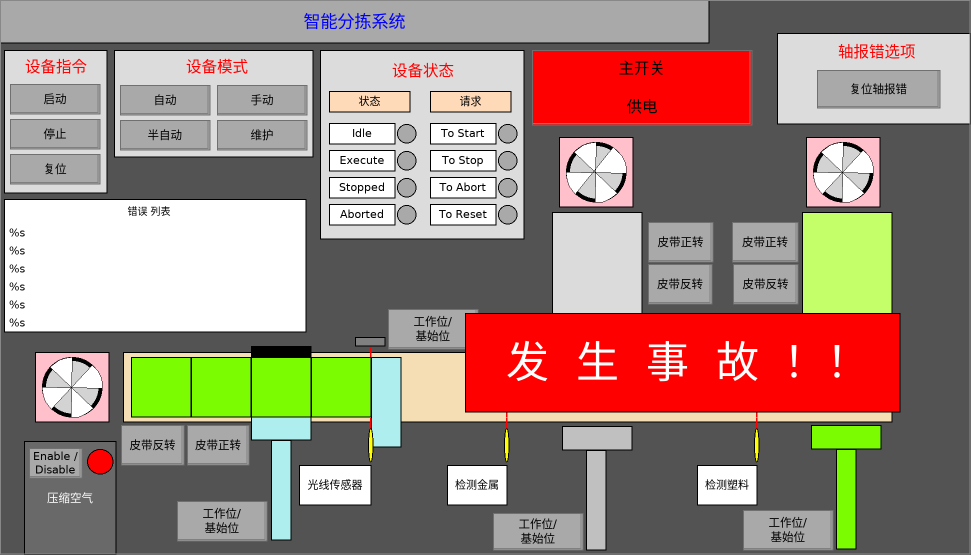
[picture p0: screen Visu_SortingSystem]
VISUALIZATION Visu_SortingSystem  // 971x555
    Rectangle (777,33 194x91)
    Rectangle (123,352 769x70)
    Rectangle (802,212 90x140)
    Rectangle (552,212 90x140)
    Rectangle (741,337 30x9)
    Rectangle (492,337 30x9)
    Ellipse (504,428 5x34)
    Ellipse (754,428 5x34)
    Group (562,426 70x124)
        p2738717112: MAIN_Simu.Simulation.fbVisu.fYMetal
        Rectangle (0,0 70x24)
        Rectangle (24,24 20x100)
    Group (812,426 70x124)
        p2738717112: MAIN_Simu.Simulation.fbVisu.fYPlastic
        Rectangle (-1,-1 70x24)
        Rectangle (24,23 20x100)
    Group (252,417 60x124)
        p2738717112: MAIN_Simu.Simulation.fbVisu.fYClamp
        Rectangle (19,23 20x100)
        Rectangle (-1,-1 60x24)
    Rectangle (131,357 60x60), colour toggle: MAIN_Simu.Simulation.fbVisu.ArrChangeColor[4]
        p3560616238: MAIN_Simu.Simulation.fbVisu.aBoxX[4]
        p2738717112: MAIN_Simu.Simulation.fbVisu.aBoxY[4]
    Rectangle (251,357 60x60), colour toggle: MAIN_Simu.Simulation.fbVisu.ArrChangeColor[2]
        p3560616238: MAIN_Simu.Simulation.fbVisu.aBoxX[2]
        p2738717112: MAIN_Simu.Simulation.fbVisu.aBoxY[2]
    Rectangle (191,357 60x60), colour toggle: MAIN_Simu.Simulation.fbVisu.ArrChangeColor[3]
        p3560616238: MAIN_Simu.Simulation.fbVisu.aBoxX[3]
        p2738717112: MAIN_Simu.Simulation.fbVisu.aBoxY[3]
    Textfield (447,465 60x40), "检测金属"
    Textfield (697,465 60x40), "检测塑料"
    Rectangle (506,418 1x10)
    Rectangle (506,347 1x70), invisible if: MAIN_Simu.Simulation.bMetalSensor
    Rectangle (756,347 1x70), invisible if: MAIN_Simu.Simulation.bPlasticSensor
    Rectangle (756,418 1x10)
    Textfield (0,0 709x43), "智能分拣系统"
    Rectangle (4,50 103x143)
    Button (10,84 90x30), "启动", colour toggle: MAIN_Simu.Simulation.fbVisu.bButtonColorStart, input disabled if: NOT MAIN_Simu.Simulation.fbVisu.bButtonColorStart AND NOT MAIN_Simu.Simulation.fbVisu.bAccident
        p573394764: MAIN_Simu.Simulation.fbVisu.nButtonColorStart
        toggle MAIN_Simu.Simulation.fbVisu.bButtonStartOut
    Button (10,119 90x30), "停止", colour toggle: MAIN_Simu.Simulation.fbVisu.bButtonColorStop, input disabled if: NOT MAIN_Simu.Simulation.fbVisu.bButtonColorStop
        p573394764: MAIN_Simu.Simulation.fbVisu.nButtonColorStop
        toggle MAIN_Simu.Simulation.fbVisu.bButtonStopOut
    Button (10,154 90x30), "复位", colour toggle: MAIN_Simu.Simulation.fbVisu.bButtonColorReset, input disabled if: NOT MAIN_Simu.Simulation.fbVisu.bButtonColorReset
        p573394764: MAIN_Simu.Simulation.fbVisu.nButtonColorReset
        toggle MAIN_Simu.Simulation.fbVisu.bButtonResetOut
    Textfield (7,54 98x25), "设备指令"
    Rectangle (114,50 199x107)
    Button (120,85 90x30), "自动", colour toggle: MAIN_Simu.Simulation.fbVisu.bButtonColorAuto, input disabled if: NOT MAIN_Simu.Simulation.fbVisu.bButtonColorAutoNew
        p573394764: MAIN_Simu.Simulation.fbVisu.nButtonColorAuto
        toggle MAIN_Simu.Simulation.fbVisu.bButtonAutoOut
    Button (217,85 90x30), "手动", colour toggle: MAIN_Simu.Simulation.fbVisu.bButtonColorManu, input disabled if: NOT MAIN_Simu.Simulation.fbVisu.bButtonColorManuNew
        p573394764: MAIN_Simu.Simulation.fbVisu.nButtonColorManu
        toggle MAIN_Simu.Simulation.fbVisu.bButtonManuOut
    Button (120,120 90x30), "半自动", colour toggle: MAIN_Simu.Simulation.fbVisu.bButtonColorSemi, input disabled if: NOT MAIN_Simu.Simulation.fbVisu.bButtonColorSemiNew
        p573394764: MAIN_Simu.Simulation.fbVisu.nButtonColorSemi
        toggle MAIN_Simu.Simulation.fbVisu.bButtonSemiOut
    Button (217,120 90x30), "维护", colour toggle: MAIN_Simu.Simulation.fbVisu.bButtonColorMaint, input disabled if: NOT MAIN_Simu.Simulation.fbVisu.bButtonColorMaintNew
        p573394764: MAIN_Simu.Simulation.fbVisu.nButtonColorMaint
        toggle MAIN_Simu.Simulation.fbVisu.bButtonMaintenanceOut
    Textfield (156,52 122x29), "设备模式"
    Rectangle (24,441 92x114), "压缩空气"
    Ellipse (87,449 26x25), colour toggle: MAIN_Simu.Simulation.fbVisu.bComprAirEnabled
    Button (648,222 65x40), "皮带正转", colour toggle: MAIN_Simu.Simulation.fbVisu.bButtonColorMetalFw, invisible if: NOT (MAIN_Simu.Simulation.fbVisu.bManual OR MAIN_Simu.Simulation.fbVisu.bMaintenance), input disabled if: NOT MAIN_Simu.Simulation.fbVisu.bButtonColorMetalFw
        p573394764: MAIN_Simu.Simulation.fbVisu.nButtonColorMetalFw
        toggle MAIN_Simu.Simulation.fbVisu.bButtonMetalFwOut
    Button (732,222 66x40), "皮带正转", colour toggle: MAIN_Simu.Simulation.fbVisu.bButtonColorPlasticFw, invisible if: NOT (MAIN_Simu.Simulation.fbVisu.bManual OR MAIN_Simu.Simulation.fbVisu.bMaintenance), input disabled if: NOT MAIN_Simu.Simulation.fbVisu.bButtonColorPlasticFw
        p573394764: MAIN_Simu.Simulation.fbVisu.nButtonColorPlasticFw
        toggle MAIN_Simu.Simulation.fbVisu.bButtonPlasticFwOut
    Button (187,425 62x40), "皮带正转", colour toggle: MAIN_Simu.Simulation.fbVisu.bButtonColorMainFw, invisible if: NOT (MAIN_Simu.Simulation.fbVisu.bManual OR MAIN_Simu.Simulation.fbVisu.bMaintenance), input disabled if: NOT MAIN_Simu.Simulation.fbVisu.bButtonColorMainFw
        p573394764: MAIN_Simu.Simulation.fbVisu.nButtonColorMainFw
        toggle MAIN_Simu.Simulation.fbVisu.bButtonMainFwOut
    Button (648,264 64x40), "皮带反转", colour toggle: MAIN_Simu.Simulation.fbVisu.bButtonColorMetalBw, invisible if: NOT (MAIN_Simu.Simulation.fbVisu.bManual OR MAIN_Simu.Simulation.fbVisu.bMaintenance), input disabled if: NOT MAIN_Simu.Simulation.fbVisu.bButtonColorMetalBw
        p573394764: MAIN_Simu.Simulation.fbVisu.nButtonColorMetalBw
        toggle MAIN_Simu.Simulation.fbVisu.bButtonMetalBwOut
    Button (733,264 65x40), "皮带反转", colour toggle: MAIN_Simu.Simulation.fbVisu.bButtonColorPlasticBw, invisible if: NOT (MAIN_Simu.Simulation.fbVisu.bManual OR MAIN_Simu.Simulation.fbVisu.bMaintenance), input disabled if: NOT MAIN_Simu.Simulation.fbVisu.bButtonColorPlasticBw
        p573394764: MAIN_Simu.Simulation.fbVisu.nButtonColorPlasticBw
        toggle MAIN_Simu.Simulation.fbVisu.bButtonPlasticBwOut
    Button (121,425 63x40), "皮带反转", colour toggle: MAIN_Simu.Simulation.fbVisu.bButtonColorMainBw, invisible if: NOT (MAIN_Simu.Simulation.fbVisu.bManual OR MAIN_Simu.Simulation.fbVisu.bMaintenance), input disabled if: NOT MAIN_Simu.Simulation.fbVisu.bButtonColorMainBw
        p573394764: MAIN_Simu.Simulation.fbVisu.nButtonColorMainBw
        toggle MAIN_Simu.Simulation.fbVisu.bButtonMainBwOut
    Button (388,309 90x40), "工作位/ 基始位", colour toggle: MAIN_Simu.Simulation.fbVisu.bButtonColorBarrier, invisible if: NOT (MAIN_Simu.Simulation.fbVisu.bManual OR MAIN_Simu.Simulation.fbVisu.bMaintenance), input disabled if: NOT MAIN_Simu.Simulation.fbVisu.bButtonColorBarrier
        p573394764: MAIN_Simu.Simulation.fbVisu.nButtonColorBarrier
        toggle MAIN_Simu.Simulation.fbVisu.bButtonBarrierToWorkOut
    Button (177,501 90x40), "工作位/ 基始位", colour toggle: MAIN_Simu.Simulation.fbVisu.bButtonColorClamp, invisible if: NOT (MAIN_Simu.Simulation.fbVisu.bManual OR MAIN_Simu.Simulation.fbVisu.bMaintenance), input disabled if: NOT MAIN_Simu.Simulation.fbVisu.bButtonColorClamp
        p573394764: MAIN_Simu.Simulation.fbVisu.nButtonColorClamp
        toggle MAIN_Simu.Simulation.fbVisu.bButtonClampToWorkOut
    Button (493,513 90x37), "工作位/ 基始位", colour toggle: MAIN_Simu.Simulation.fbVisu.bButtonColorMetalCyl, invisible if: NOT (MAIN_Simu.Simulation.fbVisu.bManual OR MAIN_Simu.Simulation.fbVisu.bMaintenance), input disabled if: NOT MAIN_Simu.Simulation.fbVisu.bButtonColorMetalCyl
        p573394764: MAIN_Simu.Simulation.fbVisu.nButtonColorMetalCyl
        toggle MAIN_Simu.Simulation.fbVisu.bButtonMetalToWorkOut
    Button (743,510 90x40), "工作位/ 基始位", colour toggle: MAIN_Simu.Simulation.fbVisu.bButtonColorPlasticCyl, invisible if: NOT (MAIN_Simu.Simulation.fbVisu.bManual OR MAIN_Simu.Simulation.fbVisu.bMaintenance), input disabled if: NOT MAIN_Simu.Simulation.fbVisu.bButtonColorPlasticCyl
        p573394764: MAIN_Simu.Simulation.fbVisu.nButtonColorPlasticCyl
        toggle MAIN_Simu.Simulation.fbVisu.bButtonPlasticToWorkOut
    Rectangle (371,357 30x90)
        p2738717112: MAIN_Simu.Simulation.fbVisu.fYBarrier
    Rectangle (355,337 30x9)
    Ellipse (368,428 5x34)
    Rectangle (370,418 1x10)
    Rectangle (370,347 1x70), invisible if: MAIN_Simu.Simulation.bBarrierSensor
    Textfield (299,465 72x40), "光线传感器"
    Button (532,50 220x75), "主开关 供电", colour toggle: MAIN_Simu.Simulation.fbVisu.bPowerEnabled
        toggle MAIN_Simu.Simulation.fbVisu.bButtonPowerOut
    Rectangle (320,50 204x189)
    Textfield (329,123 66x21), "Idle"
    Textfield (329,150 66x21), "Execute"
    Textfield (329,177 66x21), "Stopped"
    Textfield (329,204 66x21), "Aborted"
    Textfield (430,123 66x21), "To Start"
    Textfield (430,150 66x21), "To Stop"
    Textfield (430,177 66x21), "To Abort"
    Textfield (430,204 66x21), "To Reset"
    Textfield (329,91 81x21), "状态"
    Textfield (430,91 81x21), "请求"
    Ellipse (397,124 19x19), colour toggle: MAIN_Simu.Simulation.fbVisu.bIdle
    Ellipse (397,151 19x19), colour toggle: MAIN_Simu.Simulation.fbVisu.bStarted AND MAIN_Simu.Simulation.fbVisu.bPowerEnabled
    Ellipse (397,178 19x19), colour toggle: MAIN_Simu.Simulation.fbVisu.bStopped
    Ellipse (397,205 19x19), colour toggle: MAIN_Simu.Simulation.fbVisu.bAborted
    Ellipse (498,124 19x19), colour toggle: MAIN_Simu.Simulation.fbVisu.bButtonStartIn
    Ellipse (498,151 19x19), colour toggle: MAIN_Simu.Simulation.fbVisu.bButtonStopIn
    Ellipse (498,205 19x19), colour toggle: MAIN_Simu.Simulation.fbVisu.bReset
    Ellipse (498,178 19x19), colour toggle: MAIN_Simu.Simulation.fbVisu.bButtonAbortIn
    Rectangle (251,346 60x11)
    Rectangle (311,357 60x60), colour toggle: MAIN_Simu.Simulation.fbVisu.ArrChangeColor[1]
        p3560616238: MAIN_Simu.Simulation.fbVisu.aBoxX[1]
        p2738717112: MAIN_Simu.Simulation.fbVisu.aBoxY[1]
    Button (29,448 53x30), "Enable / Disable", colour toggle: MAIN_Simu.Simulation.fbVisu.bButtonColorComprAir, invisible if: NOT MAIN_Simu.Simulation.fbVisu.bMaintenance, input disabled if: NOT MAIN_Simu.Simulation.fbVisu.bButtonColorComprAir
        p573394764: MAIN_Simu.Simulation.fbVisu.nButtonColorComprAir
        toggle MAIN_Simu.Simulation.fbVisu.bButtonComprAirOut
    Rectangle (4,199 302x133)
    Textfield (76,202 146x19), "错误 列表"
    Textfield (6,225 298x16), "%s", text variable: MAIN_Simu.Simulation.fbVisu.sMessageMainAxis
    Textfield (6,243 298x16), "%s", text variable: MAIN_Simu.Simulation.fbVisu.sMessageMetalAxis
    Textfield (6,261 298x16), "%s", text variable: MAIN_Simu.Simulation.fbVisu.sMessagePlasticAxis
    Textfield (6,279 298x16), "%s", text variable: MAIN_Simu.Simulation.fbVisu.sMessageClamp
    Textfield (6,297 298x16), "%s", text variable: MAIN_Simu.Simulation.fbVisu.sMessageMetalCyl
    Textfield (6,315 298x16), "%s", text variable: MAIN_Simu.Simulation.fbVisu.sMessagePlasticCyl
    Rectangle (465,313 435x99), "发 生 事 故 ！！", invisible if: NOT MAIN_Simu.Simulation.fbVisu.bAccident
    Textfield (35,352 74x70), invisible if: BIT_TO_BOOL(MAIN_Simu.Simulation.fbVisu.MainAxisState.StateDWord.2)
    Rectangle (71,357 1x60)
    Rectangle (42,387 60x1)
    Ellipse (42,357 60x60)
    Polygon (72,357) (71,417) (78,417) (83,415) (88,412) (93,408) (50,367) (47,371) (45,375) (43,380) (42,387) (102,388) (102,382) (101,377) (98,371) (92,365) (51,409) (48,405) (45,401) (43,395) (42,388) (43,382) (44,377) (47,371) (51,366) (55,363) (59,360) (65,358)
        p2858320360: MAIN_Simu.Simulation.fbVisu.nAngleMain
    Textfield (559,137 74x70), invisible if: BIT_TO_BOOL(MAIN_Simu.Simulation.fbVisu.MetalAxisState.StateDWord.2)
    Rectangle (595,142 1x60)
    Rectangle (566,172 60x1)
    Ellipse (566,142 60x60)
    Polygon (596,142) (595,202) (602,202) (607,200) (612,197) (617,193) (574,152) (571,156) (569,160) (567,165) (566,172) (626,173) (626,167) (625,162) (622,156) (613,147) (575,194) (572,190) (569,186) (567,180) (566,173) (567,167) (568,162) (571,156) (575,151) (579,148) (583,145) (589,143)
        p2858320360: MAIN_Simu.Simulation.fbVisu.nAngleMetal
    Textfield (806,137 74x70), invisible if: BIT_TO_BOOL(MAIN_Simu.Simulation.fbVisu.PlasticAxisState.StateDWord.2)
    Rectangle (842,142 1x60)
    Rectangle (813,172 60x1)
    Ellipse (813,142 60x60)
    Polygon (843,142) (842,202) (849,202) (854,200) (859,197) (864,193) (821,152) (818,156) (816,160) (814,165) (813,172) (873,173) (873,167) (872,162) (869,156) (863,150) (822,194) (819,190) (816,186) (814,180) (813,173) (814,167) (815,162) (818,156) (822,151) (826,148) (830,145) (836,143)
        p2858320360: MAIN_Simu.Simulation.fbVisu.nAnglePlastic
    Button (817,70 123x38), "复位轴报错", input disabled if: NOT MAIN_Simu.Simulation.fbVisu.bError
        p2175578022: 16#00FFFF80
        tap MAIN_Simu.Simulation.fbVisu.bresetAxis
    Textfield (799,37 156x29), "轴报错选项"
    Textfield (362,56 122x29), "设备状态"
END_VISUALIZATION
